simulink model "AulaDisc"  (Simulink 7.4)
settings: Solver=ode45  StartTime=0.0  StopTime=10.0  MaxStep=.02  RelTol=1e-3
libraries: cstblocks x8

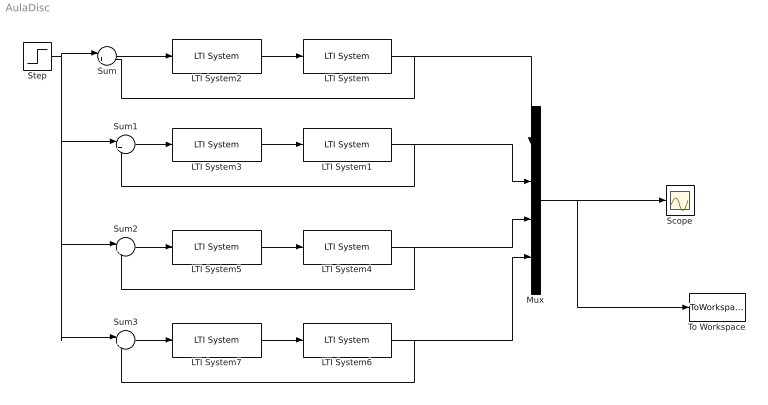
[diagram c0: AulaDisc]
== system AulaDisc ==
  LTI System : cstblocks/LTI System  SystemSampleTime=-1  sys=syss1  IC=[]
  LTI System1 : cstblocks/LTI System  SystemSampleTime=-1  sys=syss2  IC=[]
  LTI System2 : cstblocks/LTI System  SystemSampleTime=-1  sys=cs1  IC=[]
  LTI System3 : cstblocks/LTI System  SystemSampleTime=-1  sys=cs2  IC=[]
  LTI System4 : cstblocks/LTI System  SystemSampleTime=-1  sys=syss3  IC=[]
  LTI System5 : cstblocks/LTI System  SystemSampleTime=-1  sys=cs3  IC=[]
  LTI System6 : cstblocks/LTI System  SystemSampleTime=-1  sys=syss4  IC=[]
  LTI System7 : cstblocks/LTI System  SystemSampleTime=-1  sys=cs4  IC=[]
  Mux : Mux
  Scope : Scope
  Step : Step  SampleTime=0
  Sum{,1..3} (4 alike) : Sum  Inputs=|+-  OutDataType=fixdt(1, 16)  OutScaling=2^0
  To Workspace : ToWorkspace  VariableName=simout  SampleTime=-1  SaveFormat=Structure With Time
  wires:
  LTI System/1 -> Sum/2, Mux/1
  LTI System2/1 -> LTI System/1
  Sum/1 -> LTI System2/1
  Step/1 -> Sum/1, Sum1/1, Sum2/1, Sum3/1
  LTI System1/1 -> Sum1/2, Mux/2
  LTI System3/1 -> LTI System1/1
  Sum1/1 -> LTI System3/1
  LTI System4/1 -> Sum2/2, Mux/3
  LTI System5/1 -> LTI System4/1
  Sum2/1 -> LTI System5/1
  LTI System6/1 -> Sum3/2, Mux/4
  LTI System7/1 -> LTI System6/1
  Sum3/1 -> LTI System7/1
  Mux/1 -> Scope/1, To Workspace/1
